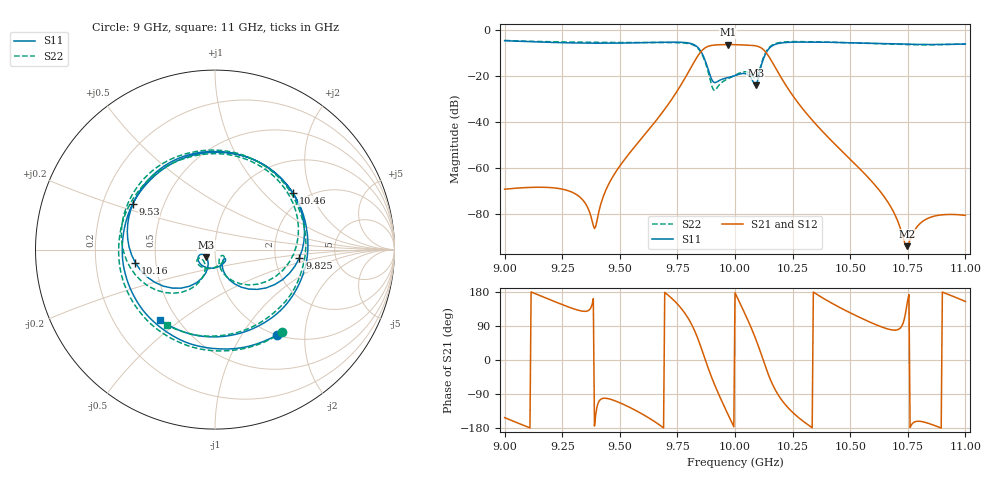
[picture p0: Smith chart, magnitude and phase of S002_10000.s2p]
# Hz S DB R 50
! Planar, S50180, , 20.4.1/1
! Date: 14.11.2021 12:36:49
! Data: Format (Calibration Info)
! Freq	S11:dB/Ang(--)	S21:dB/Ang(--)	S12:dB/Ang(--)	S22:dB/Ang(--)
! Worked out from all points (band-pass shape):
!   401 points, 9 GHz to 11 GHz, reference 50 ohm
!   highest |S21| = -6.31 dB at 9.97 GHz (marker M1); lowest = -93.9 dB at 10.74 GHz (marker M2)
!   |S21| within 3 dB of the highest: 9.853 GHz to 10.13 GHz (278 MHz wide, 2.78 % of centre)
!   lowest |S11| = -23.9 dB at 10.09 GHz (marker M3), VSWR 1.14, Z = 45.2 - j3.76 ohm
!   |S11| at or under -10 dB: 9.856 GHz to 10.13 GHz (278.5 MHz wide, 2.79 % of centre)
!   |S22| runs from -26.2 to -4.5 dB; largest |S21 - S12| = 0.00051
!   S11 on the Smith chart (normalised r, x): 9 GHz: 1.00, -1.45; 9.53 GHz: 0.33, +0.23; 9.825 GHz: 2.75, -0.32; 10.16 GHz: 0.38, -0.07; 10.46 GHz: 1.70, +1.50; 11 GHz: 0.41, -0.42
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9e9  -4.61 -54.1  -69.10 -152.1  -69.11 -152.1  -4.52 -50.7
9.225e9  -5.43 -115.5  -68.67 152.3  -68.67 152.3  -5.13 -110.2
9.335e9  -5.65 -147.6  -73.32 129.2  -73.32 129.2  -5.28 -140.9
9.4e9  -5.71 -167.4  -83.21 -126.7  -83.22 -126.7  -5.34 -159.6
9.53e9  -5.61 151.0  -55.01 -121.1  -55.01 -121.2  -5.40 160.9
9.67e9  -5.34 98.5  -37.70 -170.4  -37.71 -170.4  -5.42 110.6
9.76e9  -5.30 51.4  -24.73 141.0  -24.74 140.9  -5.52 63.5
9.825e9  -6.51 -5.5  -13.47 76.9  -13.47 76.8  -6.82 3.4
9.885e9  -17.54 -68.4  -7.01 -23.6  -7.02 -23.6  -18.70 -73.2
9.91e9  -22.79 -49.1  -6.52 -63.0  -6.53 -63.0  -26.19 -48.8
9.97e9  -20.65 -66.1  -6.31 -144.3  -6.31 -144.3  -21.16 -69.5
1e10  -19.77 -93.8  -6.34 177.4  -6.35 177.4  -19.63 -98.6
1.005e10  -19.10 -146.9  -6.54 112.9  -6.54 112.9  -18.18 -142.2
1.009e10  -23.92 -139.4  -6.87 55.5  -6.88 55.5  -21.01 -136.9
1.012e10  -13.51 -119.1  -8.21 4.2  -8.22 4.2  -12.89 -118.2
1.016e10  -6.95 -170.5  -13.65 -60.7  -13.65 -60.7  -6.62 -162.8
1.024e10  -5.30 123.9  -26.91 -132.1  -26.92 -132.1  -5.05 135.9
1.0335e10  -5.26 79.6  -39.10 -178.6  -39.11 -178.7  -5.11 93.3
1.046e10  -5.41 36.0  -52.19 136.8  -52.20 136.8  -5.40 49.5
1.067e10  -5.95 -28.0  -75.76 80.8  -75.76 80.7  -6.10 -17.6
1.0745e10  -6.12 -50.5  -93.86 141.4  -93.87 141.4  -6.31 -41.4
1.1e10  -6.06 -127.7  -80.49 154.5  -80.50 154.5  -6.05 -122.4
